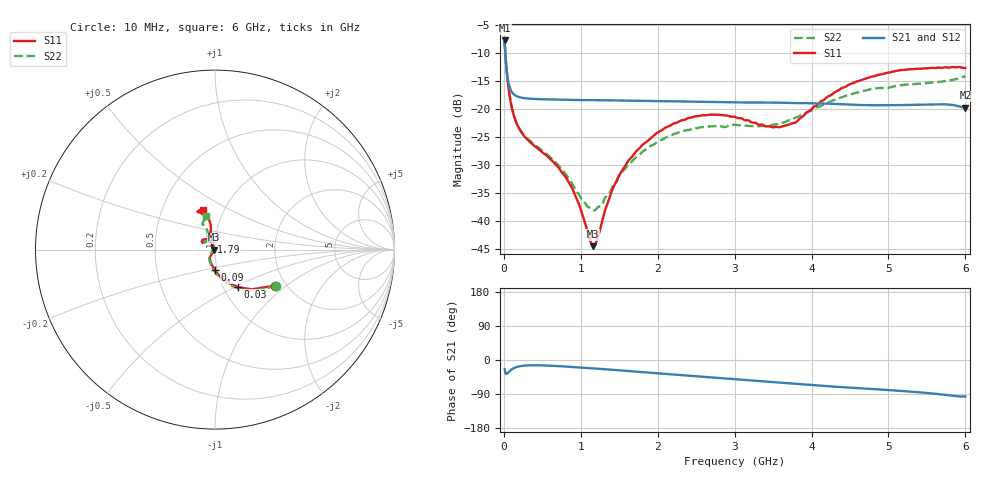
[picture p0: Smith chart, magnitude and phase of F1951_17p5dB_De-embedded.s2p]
! Integrated Device Technology
! Corporate Headquarters
! 6024 Silver Creek Valley Road
! San Jose, CA 95138  USA
! Phone:  1-408-284-8200
! Toll Free:  1-800-223-1366
! Webpage:  http://www.idt.com/
! Timing and RF Division
! 515 Groton Road, Suite 102
! Westford, MA 01886-6024
! Device:  F1951
! Description: 6-bit 0.5 dB Digital Step Attenuator
! Frequency:  100.0 -  4000.00 MHz
! Package:  4x4 mm Thin QFN Plastic Package: 24 pin
! Ports:  2 RF, 6 DC
!  Pin  1  = NC
!  Pin  2  = RF1  =  Port 1
!  Pin  3  = GND
!  Pin  4  = NC
!  Pin  5  = Serial Data Out (SDO)
!  Pin  6  = NC
!  Pin  7  = Reset Bar ( RSTb)
!  Pin  8  = Clock (CLK)
!  Pin  9  = Chip Select Bar (CSb)
!  Pin 10  = NC
!  Pin 11  = Serial Data In (SDI)
!  Pin 12  = NC
!  Pin 13  = NC
!  Pin 14  = VDD
!  Pin 15  = NC
!  Pin 16  = GND
!  Pin 17  = RF2  =  Port 2
!  Pin 18  = NC
!  Pin 19  = GND
!  Pin 20  = GND
!  Pin 21  = GND
!  Pin 22  = GND
!  Pin 23  = GND
!  Pin 24  = GND
! State:  35
! Atten State:  17.5 dB
! Voltage:  +3.30 Volts
! Current:  0.486 mA
! Data:  The device was measured on a F195X evaluation board which has
!  individual transmission lines to the RF pins.  Data was collected
!  de-embedded using a Automatic Fixture Removal [AFR] (Keysight Technologies).
!  The reference plane is the edge of the package pin.
! Misc:  Lot Code  1225BCA
!  Action Tracker AT0399
! Date Measured:  2018-09-13
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# GHz S dB R 50
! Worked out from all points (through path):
!   600 points, 10 MHz to 6 GHz, reference 50 ohm
!   highest |S21| = -7.84 dB at 10 MHz (marker M1); lowest = -19.8 dB at 6 GHz (marker M2)
!   group delay of S21, straight-line fit = 39.6 ps
!   lowest |S11| = -44.4 dB at 1.16 GHz (marker M3), VSWR 1.01, Z = 49.4 + j0.0124 ohm
!   |S11| at or under -10 dB: 18.1 MHz to end of sweep
!   |S22| runs from -38.1 to -8.0 dB; largest |S21 - S12| = 0.00026
!   S11 on the Smith chart (normalised r, x): 10 MHz: 1.75, -0.82; 30 MHz: 1.17, -0.52; 90 MHz: 0.97, -0.22; 1.79 GHz: 0.96, +0.08; 6 GHz: 0.80, +0.37
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0.01  -8.23 -31.2  -7.84 -24.6  -7.84 -24.6  -8.05 -30.9
0.03  -12.22 -58.3  -12.05 -36.4  -12.05 -36.5  -12.05 -60.0
0.06  -16.21 -78.6  -15.32 -32.6  -15.32 -32.6  -16.17 -81.0
0.09  -18.89 -90.5  -16.66 -26.7  -16.66 -26.7  -18.83 -93.6
0.15  -22.04 -105.6  -17.63 -19.7  -17.63 -19.7  -21.97 -108.9
0.25  -24.59 -118.0  -18.07 -15.2  -18.07 -15.1  -24.51 -122.6
0.72  -30.64 -123.9  -18.37 -16.3  -18.37 -16.3  -30.27 -136.6
0.88  -33.95 -124.4  -18.41 -18.3  -18.41 -18.3  -33.17 -141.4
1.01  -38.32 -130.4  -18.45 -20.1  -18.45 -20.1  -36.01 -151.0
1.16  -44.45 178.8  -18.47 -22.1  -18.47 -22.1  -37.97 -178.5
1.21  -43.37 149.3  -18.47 -22.8  -18.47 -22.8  -37.67 168.9
1.44  -33.52 113.2  -18.52 -26.3  -18.52 -26.3  -33.57 136.5
1.79  -26.58 117.0  -18.57 -31.7  -18.57 -31.7  -27.80 128.6
2.01  -24.14 124.2  -18.63 -35.2  -18.63 -35.2  -25.74 131.8
2.49  -21.33 138.8  -18.74 -42.8  -18.74 -42.8  -23.47 140.2
3.01  -21.46 150.0  -18.86 -50.8  -18.86 -50.7  -22.84 144.1
3.58  -23.28 129.4  -18.91 -59.5  -18.91 -59.5  -22.60 126.2
3.79  -22.46 113.1  -18.98 -62.7  -18.99 -62.7  -21.58 119.2
4.01  -19.89 103.6  -19.01 -66.1  -19.01 -66.0  -20.19 113.9
4.49  -15.67 100.8  -19.24 -73.1  -19.24 -73.0  -17.49 112.8
5.01  -13.55 109.5  -19.37 -79.4  -19.37 -79.3  -16.23 115.9
6  -12.73 107.0  -19.81 -96.3  -19.81 -96.2  -14.19 105.0
